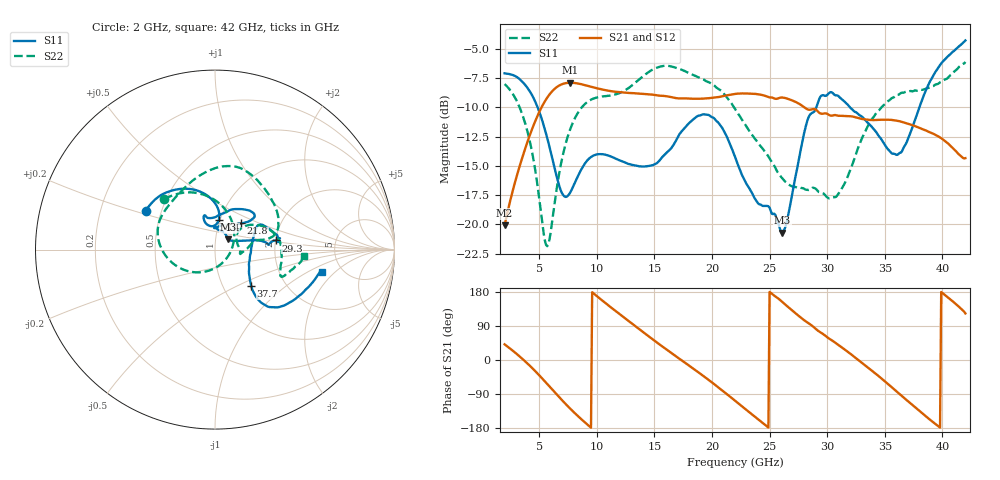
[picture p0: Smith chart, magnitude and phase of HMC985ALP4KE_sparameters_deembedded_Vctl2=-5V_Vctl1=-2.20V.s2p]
!s2p File: Measurements: S11, S21, S12, S22
# GHz S dB R 50.0
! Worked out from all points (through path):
!   401 points, 2 GHz to 42 GHz, reference 50 ohm
!   highest |S21| = -7.89 dB at 7.7 GHz (marker M1); lowest = -20.1 dB at 2 GHz (marker M2)
!   lowest |S11| = -20.7 dB at 26.1 GHz (marker M3), VSWR 1.20, Z = 57.4 + j6.64 ohm
!   |S11| at or under -10 dB: 4.869 GHz to 29.06 GHz (24.19 GHz wide, 143 % of centre); 31.99 GHz to 38 GHz (6.016 GHz wide, 17.2 % of centre)
!   |S22| runs from -21.9 to -6.1 dB; largest |S21 - S12| = 0.00048
!   S11 on the Smith chart (normalised r, x): 2 GHz: 0.41, +0.22; 6.4 GHz: 0.99, +0.34; 21.8 GHz: 1.27, +0.39; 29.3 GHz: 2.01, +0.23; 37.7 GHz: 1.35, -0.60; 42 GHz: 3.52, -1.43
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2  -7.08 150.8  -20.07 41.3  -20.07 41.3  -8.00 135.3
4  -8.35 117.5  -12.89 -9.7  -12.90 -9.7  -12.12 81.2
5.6  -12.25 87.8  -9.31 -59.9  -9.31 -59.9  -21.75 -26.5
6.4  -15.44 82.6  -8.36 -86.8  -8.37 -86.8  -17.76 -111.0
7.7  -17.26 103.8  -7.89 -128.5  -7.89 -128.5  -11.85 -165.1
8.7  -15.22 110.4  -8.03 -157.4  -8.03 -157.4  -9.99 171.5
10.3  -13.99 106.9  -8.43 161.3  -8.43 161.3  -9.09 148.2
12.3  -14.63 104.3  -8.73 113.7  -8.73 113.7  -8.62 123.2
15.4  -14.59 86.7  -8.99 42.2  -9.00 42.2  -6.54 81.3
18.4  -11.00 51.9  -9.26 -23.3  -9.26 -23.3  -7.24 49.1
21.8  -13.70 45.2  -8.87 -102.4  -8.88 -102.4  -9.81 12.4
22  -14.21 47.8  -8.85 -107.4  -8.86 -107.4  -10.12 11.8
24.1  -18.27 88.6  -8.89 -158.7  -8.89 -158.7  -13.17 11.6
26.1  -20.70 38.4  -9.15 153.4  -9.16 153.4  -16.05 -3.9
28.7  -10.46 5.0  -10.15 90.2  -10.16 90.2  -16.88 -5.2
29.3  -9.31 8.6  -10.45 75.2  -10.45 75.2  -17.24 -1.0
30.9  -8.98 13.2  -10.70 41.1  -10.70 41.1  -17.49 26.2
32.4  -10.37 25.9  -10.83 7.3  -10.83 7.3  -14.29 38.9
35.4  -13.69 6.7  -11.06 -66.5  -11.06 -66.4  -9.39 16.0
37.7  -10.88 -45.1  -11.62 -126.6  -11.62 -126.5  -8.55 -6.3
39.7  -6.51 -42.9  -12.50 -175.9  -12.50 -175.9  -7.93 -22.3
42  -4.28 -12.0  -14.33 122.9  -14.34 122.9  -6.11 -4.1
